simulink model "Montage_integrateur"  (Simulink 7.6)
settings: Solver=ode23t  StartTime=0.0  StopTime=2.4  RelTol=1e-3
StopFcn:
  | close all
  | load signaux_integrateur.mat
  | plot(x(1,:),x(2,:))
  | hold on
  | plot(x(1,:),x(3,:))
  | axis([0 2.4 -2 6])
  | grid
  | title('Montage intégrateur')
  | xlabel('temps')
  | delete *.mat
libraries: powerlib x19

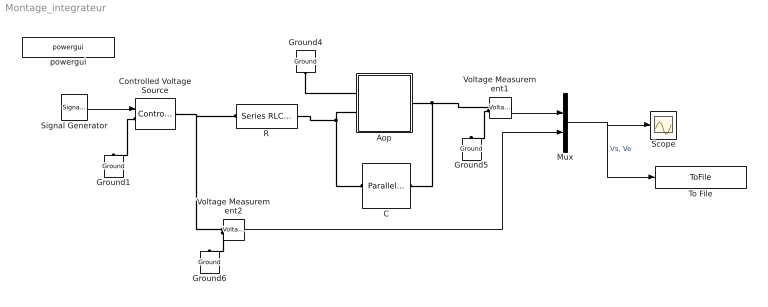
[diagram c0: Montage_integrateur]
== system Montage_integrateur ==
  Aop : Subsystem
  C : powerlib/Elements/Parallel RLC Branch  DialogController=POWERSYS.PowerSysDialog  PhysicalDomain=powersysdomain  SubClassName=unknown  LeftPortType=p1  RightPortType=p1  LConnTagsString=a  RConnTagsString=__new0  BranchType=C  Resistance=1  Inductance=1e-3  SetiL0=off  InitialCurrent=0  Capacitance=1e-6  Setx0=off  InitialVoltage=0  Measurements=Branch voltage and current
  Controlled Voltage Source : powerlib/Electrical Sources/Controlled Voltage Source  DialogController=POWERSYS.PowerSysDialog  SystemSampleTime=-1  Initialize=on  Source_Type=AC  Amplitude=0  Phase=0  Frequency=0  Measurements=None
  Ground{1,4..6} (4 alike) : powerlib/Elements/Ground  DialogController=POWERSYS.PowerSysDialog  PhysicalDomain=powersysdomain  SubClassName=unknown  LeftPortType=p1  RightPortType=p1  LConnTagsString=a
  Mux : Mux  Inputs=2
  R : powerlib/Elements/Series RLC Branch  DialogController=POWERSYS.PowerSysDialog  PhysicalDomain=powersysdomain  SubClassName=unknown  LeftPortType=p1  RightPortType=p1  LConnTagsString=__new0  RConnTagsString=__new0  BranchType=R  Resistance=100e3  Inductance=10e-3  SetiL0=off  InitialCurrent=0  Capacitance=0  Setx0=off  InitialVoltage=0  Measurements=None
  Scope : Scope
  Signal Generator : SignalGenerator  WaveForm=square
  To File : ToFile  Filename=signaux_integrateur  MatrixName=x
  Voltage Measurement1 : powerlib/Measurements/Voltage Measurement  DialogController=POWERSYS.PowerSysDialog  SystemSampleTime=-1  PhasorSimulation=off  OutputType=Complex  PSBequivalent=0
  Voltage Measurement2 : powerlib/Measurements/Voltage Measurement  DialogController=POWERSYS.PowerSysDialog  SystemSampleTime=-1  PhasorSimulation=off  OutputType=Complex  PSBequivalent=0
  powergui : powerlib/powergui  Priority=1  SystemSampleTime=-1  SimulationMode=Continuous  SampleTime=50e-6  frequency=60  SPID=off  DisableSnubberDevices=off  DisableRonSwitches=off  DisableVfSwitches=off  SwTol=0  Interpol=off  frequencyindice=0  echomessages=off  HookPort=off  DisplayEquations=off  FunctionMessages=off  EnableUseOfTLC=off  x0status=blocks  RestoreLinks=warning  ResistiveCurrentMeasurement=off  Ylog=off  Xlog=on  ShowGrid=off  save=off  variable=ZData  ZoomFFT=off  StartTime=0.0  cycles=1  DisplayStyle=1  fundamental=60  FreqAxis=off  MaxFrequency=1000  frequencyindicesteady=1  display=off  methode=off
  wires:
  Voltage Measurement1/1 -> Mux/1
  Mux/1 -> Scope/1, To File/1  "Vs, Ve"
  Voltage Measurement2/1 -> Mux/2
  Signal Generator/1 -> Controlled Voltage Source/1
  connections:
  Ground4/LConn1 -- Aop/LConn1
  C/RConn1 -- Voltage Measurement1/LConn1 -- Aop/RConn1
  C/LConn1 -- Aop/LConn2 -- R/RConn1
  Voltage Measurement1/LConn2 -- Ground5/LConn1
  Controlled Voltage Source/RConn1 -- Voltage Measurement2/LConn1 -- R/LConn1
  Voltage Measurement2/LConn2 -- Ground6/LConn1
  Controlled Voltage Source/LConn1 -- Ground1/LConn1

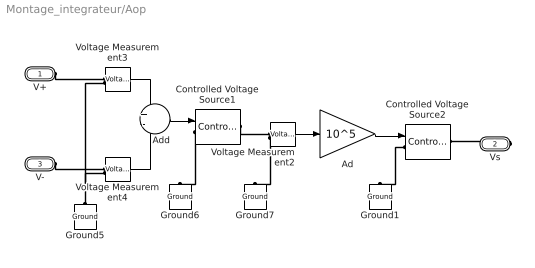
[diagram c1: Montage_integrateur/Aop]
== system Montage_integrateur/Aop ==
  Ad : Gain  Gain=10^5
  Add : Sum  Inputs=+-
  Controlled Voltage Source1 : powerlib/Electrical Sources/Controlled Voltage Source  DialogController=POWERSYS.PowerSysDialog  SystemSampleTime=-1  Initialize=on  Source_Type=AC  Amplitude=0  Phase=0  Frequency=0  Measurements=None
  Controlled Voltage Source2 : powerlib/Electrical Sources/Controlled Voltage Source  DialogController=POWERSYS.PowerSysDialog  SystemSampleTime=-1  Initialize=on  Source_Type=AC  Amplitude=0  Phase=0  Frequency=0  Measurements=None
  Ground{1,5..7} (4 alike) : powerlib/Elements/Ground  DialogController=POWERSYS.PowerSysDialog  PhysicalDomain=powersysdomain  SubClassName=unknown  LeftPortType=p1  RightPortType=p1  LConnTagsString=a
  Voltage Measurement2 : powerlib/Measurements/Voltage Measurement  DialogController=POWERSYS.PowerSysDialog  SystemSampleTime=-1  PhasorSimulation=off  OutputType=Complex  PSBequivalent=0
  Voltage Measurement3 : powerlib/Measurements/Voltage Measurement  DialogController=POWERSYS.PowerSysDialog  SystemSampleTime=-1  PhasorSimulation=off  OutputType=Complex  PSBequivalent=0
  Voltage Measurement4 : powerlib/Measurements/Voltage Measurement  DialogController=POWERSYS.PowerSysDialog  SystemSampleTime=-1  PhasorSimulation=off  OutputType=Complex  PSBequivalent=0
  V+ : PMIOPort  Port=1  Side=Left
  Vs : PMIOPort  Port=2  Side=Right
  V- : PMIOPort  Port=3  Side=Left
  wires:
  Ad/1 -> Controlled Voltage Source2/1
  Voltage Measurement3/1 -> Add/1
  Voltage Measurement4/1 -> Add/2
  Voltage Measurement2/1 -> Ad/1
  Add/1 -> Controlled Voltage Source1/1
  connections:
  V-/RConn1 -- Voltage Measurement4/LConn1
  Vs/RConn1 -- Controlled Voltage Source2/RConn1
  V+/RConn1 -- Voltage Measurement3/LConn1
  Voltage Measurement2/LConn2 -- Ground7/LConn1
  Ground5/LConn1 -- Voltage Measurement4/LConn2 -- Voltage Measurement3/LConn2
  Controlled Voltage Source2/LConn1 -- Ground1/LConn1
  Controlled Voltage Source1/RConn1 -- Voltage Measurement2/LConn1
  Controlled Voltage Source1/LConn1 -- Ground6/LConn1
